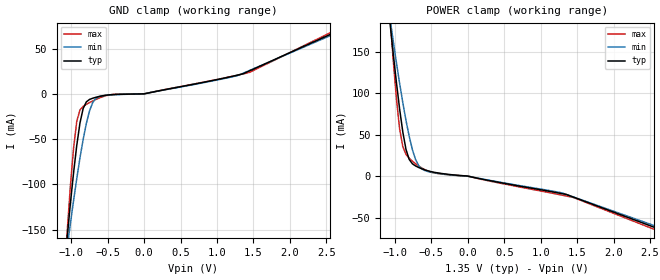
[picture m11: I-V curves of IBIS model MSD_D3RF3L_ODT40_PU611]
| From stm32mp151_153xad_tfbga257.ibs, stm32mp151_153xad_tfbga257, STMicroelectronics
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[Model] MSD_D3RF3L_ODT40_PU611
Model_type   Input
C_comp 2.379pF   2.339pF   2.433pF
Vinh = 810.000mV
Vinl = 540.000mV
[Temperature Range]   25.000   125.000   -40.000
[Voltage Range]   1.350V   1.283V   1.450V
[GND Clamp Reference]   0.00V   0.00V   0.00V
[POWER Clamp Reference]   1.350V   1.283V   1.450V
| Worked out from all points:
|   GND clamp passes 1 mA (typ) near -0.46 V on its own axis
|   POWER clamp passes 1 mA (typ) near -0.14 V on its own axis
[GND Clamp]
-1.318V   -415.8mA   -341.7mA   -533.9mA
-1.055V   -159.5mA   -170.7mA   -153.7mA
-1.011V   -121.9mA   -143.9mA   -102.9mA
-966.7mV  -87.43mA   -118.1mA   -60.17mA
-922.7mV  -56.97mA   -93.68mA   -30.48mA
-878.8mV  -32.29mA   -70.85mA   -17.81mA
-834.9mV  -16.13mA   -50.29mA   -13.82mA
-747mV    -6.166mA   -18.67mA   -9.638mA
-615.1mV  -2.932mA   -2.91mA    -4.606mA
200nV     3.403nA    3.263nA    3.449nA
1.45V     25.52mA    25.92mA    23.83mA
2.68V     70.21mA    68.65mA    72.55mA
[Power Clamp]
-1.33V    441.5mA    364mA      566.6mA
-1.067V   185.5mA    190.6mA    192.9mA
-1.023V   148.2mA    163.4mA    140.6mA
-978.8mV  113.2mA    137.1mA    93.82mA
-934.9mV  81.06mA    112mA      57.02mA
-890.9mV  53.15mA    88.53mA    35.52mA
-847mV    32.05mA    66.96mA    26.18mA
-759.1mV  14.85mA    31.74mA    17.95mA
-671.2mV  10.28mA    12.34mA    12.03mA
-583.3mV  7.305mA    6.509mA    7.504mA
1.438V    -25.03mA   -24.88mA   -25.64mA
2.668V    -65.41mA   -63.24mA   -68.17mA
